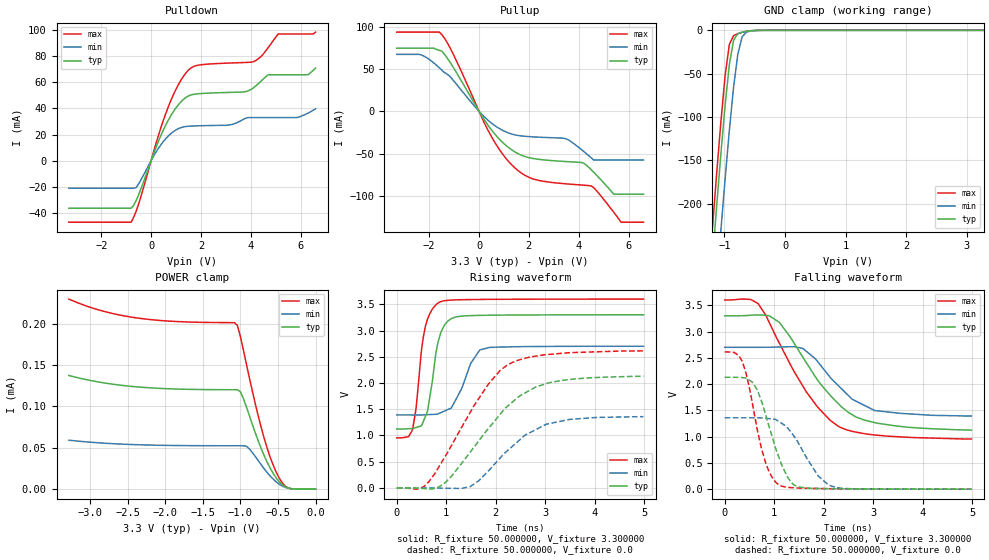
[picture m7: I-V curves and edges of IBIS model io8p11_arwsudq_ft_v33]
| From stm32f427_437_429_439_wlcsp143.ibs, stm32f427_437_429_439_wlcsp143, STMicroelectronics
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|   Model io8p11_arwsudq_ft_v33
[Model]  io8p11_arwsudq_ft_v33
Model_type I/O
Polarity   Non-Inverting
Enable   Active-Low
Vinl =   0.990000V
Vinh =   2.310000V
Vmeas =  1.650000V
Cref =   30.000000pF
Rref =   100.000000M
Vref =   0.0V
C_comp   2.911600pF   2.826600pF   2.988000pF
[Temperature Range]   25.000000   0.125000k   -40.000000
[Pullup Reference]   3.300000V   2.700000V   3.600000V
[Pulldown Reference]   0.0V   0.0V   0.0V
[POWER Clamp Reference]   3.300000V   2.700000V   3.600000V
[GND Clamp Reference]   0.0V   0.0V   0.0V
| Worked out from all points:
|   slope of the pulldown table from 0 to 0.495 V, typ, clamps not added: 20.9 ohm
|   slope of the pullup table from 0 to 0.495 V, typ, clamps not added: 22.6 ohm
|   GND clamp passes 1 mA (typ) near -0.62 V on its own axis
|   rising waveform, R_fixture 50.000000, V_fixture 3.300000: 20-80 % time 222ps typ, 364ps min, 192ps max; typ from 1.12 V to 3.3 V
|   rising waveform, R_fixture 50.000000, V_fixture 0.0: 20-80 % time 1.14ns typ, 961ps min, 1.02ns max; typ from 0 V to 2.13 V
|   falling waveform, R_fixture 50.000000, V_fixture 3.300000: 20-80 % time 1.02ns typ, 831ps min, 1ns max; typ from 3.3 V to 1.12 V
|   falling waveform, R_fixture 50.000000, V_fixture 0.0: 20-80 % time 438ps typ, 539ps min, 360ps max; typ from 2.13 V to 0 V
[Pulldown]
|Voltage   I(typ)   I(min)   I(max)
-3.3V     -36.38mA   -21.07mA   -47.08mA
-800mV    -36.38mA   -21.07mA   -47.08mA
-600mV    -30.5mA    -20.54mA   -38.69mA
700mV     31.4mA     19.11mA    41.71mA
1.2V      45.15mA    25.37mA    61.75mA
1.6V      50.35mA    26.5mA     71.06mA
3.1V      52.28mA    27.26mA    74.76mA
4.1V      55.71mA    33.02mA    75.8mA
4.7V      65.8mA     33.02mA    86.64mA
5.1V      65.8mA     33.02mA    97.03mA
6.3V      65.87mA    36.5mA     97.03mA
6.6V      70.93mA    39.72mA    98.49mA
[Pullup]
|Voltage   I(typ)   I(min)   I(max)
-3.3V     74.74mA    67.41mA    93.79mA
-2.3V     74.74mA    66.57mA    93.79mA
-1.5V     71.46mA    49mA       91.15mA
500mV     -22.07mA   -14mA      -30.03mA
1.6V      -50.64mA   -28.81mA   -70.96mA
2.3V      -56.49mA   -30.48mA   -81.16mA
3.5V      -59.53mA   -32.66mA   -85.92mA
4.2V      -61.45mA   -47.47mA   -87.46mA
4.5V      -69.1mA    -55.02mA   -88.4mA
5.4V      -98.1mA    -57.7mA    -119.3mA
5.7V      -98.1mA    -57.7mA    -131.3mA
6.6V      -98.1mA    -57.7mA    -131.3mA
[GND_clamp]
|Voltage   I(typ)   I(min)   I(max)
-3.3V     -2.32A     -2.397A    -2.297A
-1.2V     -266.4mA   -356.3mA   -229.4mA
-1.13V    -203.6mA   -293.1mA   -166.3mA
-1.06V    -143.2mA   -231.4mA   -106.2mA
-990mV    -86.95mA   -171.8mA   -52.65mA
-920mV    -39.66mA   -115.8mA   -16.36mA
-850mV    -11.49mA   -65.84mA   -6.11mA
-780mV    -3.834mA   -27.59mA   -3.88mA
-710mV    -2.09mA    -7.753mA   -2.381mA
-640mV    -1.147mA   -2.129mA   -1.22mA
-570mV    -523.9uA   -800uA     -476.8uA
3.28V     0A         0A         0A
[POWER_clamp]
|Voltage   I(typ)   I(min)   I(max)
-3.28V    137.3uA    59.14uA    229.6uA
-2.36V    123.4uA    53.65uA    206.6uA
-1.08V    120.1uA    52.41uA    201.1uA
-1.04V    120uA      52.41uA    198uA
-1V       117.7uA    52.4uA     184.5uA
-920mV    99.46uA    51.91uA    151.2uA
-720mV    48.42uA    29.12uA    73.51uA
-600mV    24.82uA    15.47uA    37.72uA
-520mV    13.1uA     8.45uA     19.84uA
-440mV    5.058uA    3.61uA     7.276uA
-360mV    1.193uA    1.129uA    1.311uA
0V        0A         0A         0A
[Ramp]
| variable   typ   min   max
dV/dt_r  1.26600/1.13918n   0.80898/0.95675n   1.56228/1.02327n
dV/dt_f  1.28238/1.01198n   0.77526/0.81952n   1.57223/1.00141n
R_load = 50.000000
[Rising Waveform]
R_fixture= 50.000000
V_fixture= 3.300000
V_fixture_min= 2.700000
V_fixture_max= 3.600000
|time   V(typ)   V(min)   V(max)
0s        1.124V     1.392V     954.3mV
320.3ps   1.132V     1.392V     1.117V
390.4ps   1.152V     1.391V     1.524V
500.5ps   1.185V     1.392V     2.634V
620.6ps   1.461V     1.397V     3.214V
850.9ps   2.835V     1.419V     3.533V
1.101ns   3.225V     1.523V     3.579V
1.491ns   3.283V     2.369V     3.59V
1.682ns   3.288V     2.632V     3.592V
4.985ns   3.3V       2.7V       3.599V
[Rising Waveform]
R_fixture= 50.000000
V_fixture= 0.0
V_fixture_min= 0.0
V_fixture_max= 0.0
|time   V(typ)   V(min)   V(max)
0s        214.5uV    83.22uV    611uV
550.6ps   -11.27mV   -120.3uV   29.39mV
951ps     78.66mV    -4.053mV   559.1mV
1.481ns   679.7mV    25.49mV    1.437V
1.852ns   1.134V     325.5mV    1.98V
2.232ns   1.554V     707.3mV    2.34V
2.593ns   1.811V     1.007V     2.472V
3.023ns   1.989V     1.215V     2.54V
3.493ns   2.067V     1.306V     2.578V
4.985ns   2.129V     1.359V     2.612V
[Falling Waveform]
R_fixture= 50.000000
V_fixture= 3.300000
V_fixture_min= 2.700000
V_fixture_max= 3.600000
|time   V(typ)   V(min)   V(max)
0s        3.3V       2.7V       3.599V
530.5ps   3.31V      2.7V       3.608V
670.7ps   3.316V     2.7V       3.534V
1.101ns   3.178V     2.705V     2.785V
1.582ns   2.509V     2.677V     1.957V
1.872ns   2.084V     2.435V     1.568V
2.302ns   1.62V      1.966V     1.192V
2.573ns   1.419V     1.714V     1.102V
3.033ns   1.266V     1.496V     1.031V
4.985ns   1.124V     1.392V     954.3mV
[Falling Waveform]
R_fixture= 50.000000
V_fixture= 0.0
V_fixture_min= 0.0
V_fixture_max= 0.0
|time   V(typ)   V(min)   V(max)
0s        2.129V     1.359V     2.612V
350.4ps   2.124V     1.358V     2.441V
560.6ps   2.031V     1.358V     1.626V
660.7ps   1.887V     1.357V     1.123V
830.8ps   1.405V     1.349V     490.5mV
1.101ns   591.7mV    1.284V     81.04mV
1.401ns   81.58mV    1.007V     26.05mV
1.882ns   13.3mV     261.1mV    12.73mV
2.102ns   9.526mV    76.73mV    9.997mV
4.985ns   214.5uV    83.22uV    611uV
